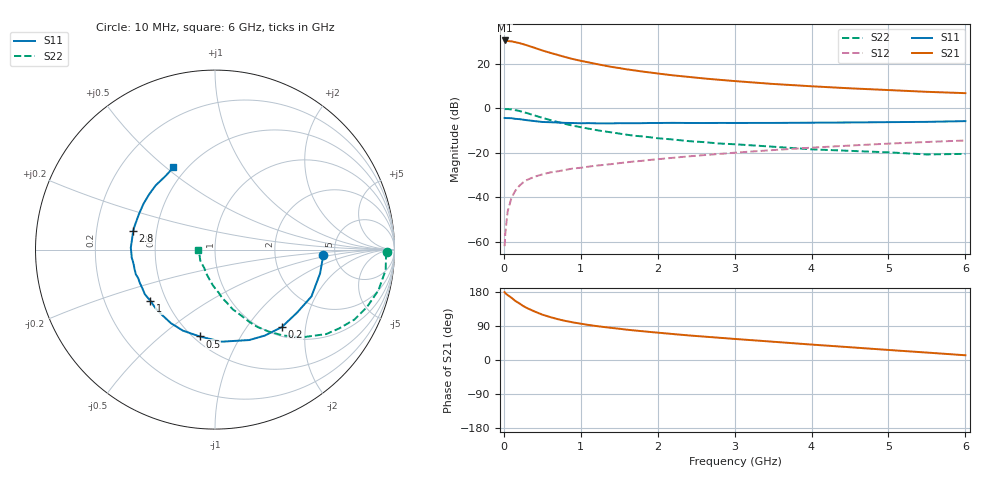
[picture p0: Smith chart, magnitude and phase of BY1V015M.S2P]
! SIEMENS Small Signal Semiconductors
! BFY420
! Si NPN RF SIEGET Grounded Emitter Transistor in MICRO-X
! VCE = 1 V  IC = 15 mA
! Common Emitter S-Parameters:  October  1996
# GHz  S  MA  R  50
!  f  S11  S21  S12  S22
! GHz  MAG  ANG  MAG  ANG  MAG  ANG  MAG  ANG
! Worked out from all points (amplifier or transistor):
!   36 points, 10 MHz to 6 GHz, reference 50 ohm
!   highest |S21| = 30.4 dB at 10 MHz (marker M1)
!   |S21| within 3 dB of that: start of sweep to 373.3 MHz
!   unconditionally stable (mu >= 1): 2.026 GHz to end of sweep
!   at 250 MHz: K = 0.25, MSG = 31.1 dB, |S12| = -33.4 dB
!   at 1.4 GHz: K = 0.88, MSG = 21.8 dB, |S12| = -25.1 dB
!   at 6 GHz: K = 1.10, MAG = 8.7 dB, |S12| = -14.5 dB
!   S11 on the Smith chart (normalised r, x): 10 MHz: 4.00, -0.41; 200 MHz: 1.16, -1.49; 500 MHz: 0.54, -0.69; 1 GHz: 0.41, -0.30; 2.8 GHz: 0.37, +0.10; 6 GHz: 0.43, +0.53
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0.01  0.6038 -3.1  33.22 179.0  0.0008 91.4  0.9575 -0.9
0.02  0.6014 -5.5  33.05 176.1  0.0016 88.0  0.9537 -2.4
0.05  0.6003 -12.8  32.26 171.3  0.0049 85.5  0.9577 -6.8
0.1  0.5975 -25.9  31.7 164.1  0.0098 79.3  0.9383 -14.0
0.15  0.5765 -37.5  30.35 155.8  0.0141 73.4  0.9053 -20.7
0.2  0.5699 -49.3  29.07 149.6  0.018 69.5  0.8695 -26.6
0.25  0.5536 -59.9  27.46 142.8  0.0215 66.3  0.8203 -32.3
0.3  0.5389 -69.2  25.85 137.1  0.0245 62.7  0.7784 -37.2
0.4  0.5144 -86.0  22.72 128.0  0.029 58.3  0.6878 -45.3
0.5  0.4914 -100.0  19.8 119.7  0.0327 54.9  0.6095 -51.7
0.6  0.4857 -111.6  17.59 113.4  0.0361 53.4  0.5441 -56.9
0.7  0.4779 -120.9  15.73 107.8  0.0383 51.7  0.4911 -61.3
0.8  0.4686 -129.1  14.05 103.2  0.0413 50.6  0.4434 -64.8
1  0.4595 -141.5  11.58 95.8  0.046 50.6  0.375 -70.2
1.1  0.4633 -147.5  10.71 92.5  0.0488 49.9  0.3484 -73.3
1.6  0.4612 -166.5  7.457 80.0  0.0612 50.0  0.2542 -83.6
2.2  0.4693 178.8  5.471 68.5  0.0772 48.9  0.1986 -93.5
2.8  0.4673 167.4  4.348 58.7  0.0942 46.5  0.1615 -102.6
3.5  0.4675 155.3  3.506 48.2  0.115 42.5  0.1368 -112.3
4.5  0.479 140.0  2.798 33.7  0.1451 34.6  0.1104 -128.2
5.5  0.494 123.9  2.335 19.6  0.1748 25.1  0.0917 -159.5
6  0.5134 116.8  2.179 12.5  0.1886 20.2  0.0944 -178.3
